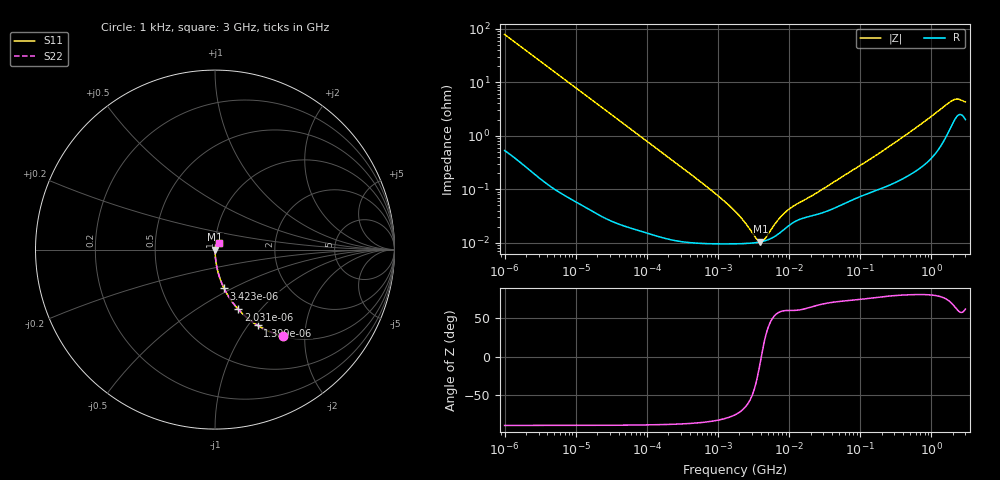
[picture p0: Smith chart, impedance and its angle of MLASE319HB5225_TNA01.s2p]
! MLASE319HB5225_TNA01  S-PARAMETER MODEL  ( Standard Model )
! Model Generated by TAIYO YUDEN Corporation (http://www.ty-top.com)
! Version 1.0
! TAIYO YUDEN Control No. 220601
! Copyright(c) 2008 TAIYO YUDEN CO.,LTD. All Rights Reserved.
! Product Description (link to TY-COMPAS)
! https://ds.yuden.co.jp/TYCOMPAS/or/detail?pn=MLASE319HB5225KTNA01&u=M
! Products Name : Multilayer Ceramic Capacitors
! Characteristics :
!  Capacitance : 2.2 [uF] , Rated Voltage : 16 [V] , TCC : B / X5R
!  Case Size : 3.2 x 1.6 / 0.126 x 0.063 [mm/inch] , Thickness : 0.85 / 0.033 [mm/inch]
!  (Conditions: Temperature = 25 [degC] , DC Bias Voltage = 0 [V])
! External Node Assignments :
!  1  o---| |---o  2
! GND o---------o GND
! Frequency Range : 1kHz  -  3GHz  [ 401 STEP ]
# MHZ S RI R 50
! Freq[MHz].  S11 Real  S11 Imag  S21 Real  S21 Imag  S12 Real  S12 Imag  S22 Real  S22 Imag
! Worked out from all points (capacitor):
!   401 points, 1 kHz to 3 GHz, reference 50 ohm
!   read as one part in series: C = 2.04 uF near 1.077 kHz
!   lowest |Z| = 10.5 mohm at 3.934 MHz (marker M1)
!   series resonance near 4.059 MHz, so ESL is about 750 pH
!   S11 on the Smith chart (normalised r, x): 1 kHz: 1.01, -1.55; 1.399 kHz: 1.01, -1.11; 2.031 kHz: 1.01, -0.77; 3.423 kHz: 1.00, -0.46; 3 GHz: 1.04, +0.08
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0.001  0.3775 -0.4814  0.6225 0.4814  0.6225 0.4814  0.3775 -0.4814
0.001399  0.2382 -0.4226  0.7618 0.4226  0.7618 0.4226  0.2382 -0.4226
0.002031  0.1303 -0.3333  0.8697 0.3333  0.8697 0.3333  0.1303 -0.3333
0.003423  0.0508 -0.2165  0.9492 0.2165  0.9492 0.2165  0.0508 -0.2165
0.006215  0.0164 -0.1238  0.9836 0.1238  0.9836 0.1238  0.0164 -0.1238
0.01216  0.00465 -0.0642  0.9954 0.0642  0.9954 0.0642  0.00465 -0.0642
0.033275  0.000808 -0.0237  0.9992 0.0237  0.9992 0.0237  0.000808 -0.0237
0.147855  0.000159 -0.00537  0.9998 0.00537  0.9998 0.00537  0.000159 -0.00537
0.791611  9.72e-05 -0.000971  0.9999 0.000971  0.9999 0.000971  9.72e-05 -0.000971
1.732051  9.6e-05 -0.000379  0.9999 0.000379  0.9999 0.000379  9.6e-05 -0.000379
2.334012  9.71e-05 -0.000231  0.9999 0.000231  0.9999 0.000231  9.71e-05 -0.000231
3.388684  0.000101 -7.23e-05  0.9999 7.23e-05  0.9999 7.23e-05  0.000101 -7.23e-05
3.93371  0.000104 -1.25e-05  0.9999 1.25e-05  0.9999 1.25e-05  0.000104 -1.25e-05
4.566395  0.000109 4.75e-05  0.9999 -4.75e-05  0.9999 -4.75e-05  0.000109 4.75e-05
6.629817  0.000138 0.000203  0.9999 -0.000203  0.9999 -0.000203  0.000138 0.000203
8.933959  0.000188 0.000329  0.9998 -0.000329  0.9998 -0.000329  0.000188 0.000329
11.59828  0.000243 0.000426  0.9998 -0.000426  0.9998 -0.000426  0.000243 0.000426
21.06097  0.000321 0.000693  0.9997 -0.000693  0.9997 -0.000693  0.000321 0.000693
256.0921  0.00123 0.0062  0.9988 -0.0062  0.9988 -0.0062  0.00123 0.0062
1917.819  0.0168 0.0405  0.9832 -0.0405  0.9832 -0.0405  0.0168 0.0405
2310.849  0.0245 0.0405  0.9755 -0.0405  0.9755 -0.0405  0.0245 0.0405
3000  0.021 0.0365  0.979 -0.0365  0.979 -0.0365  0.021 0.0365
